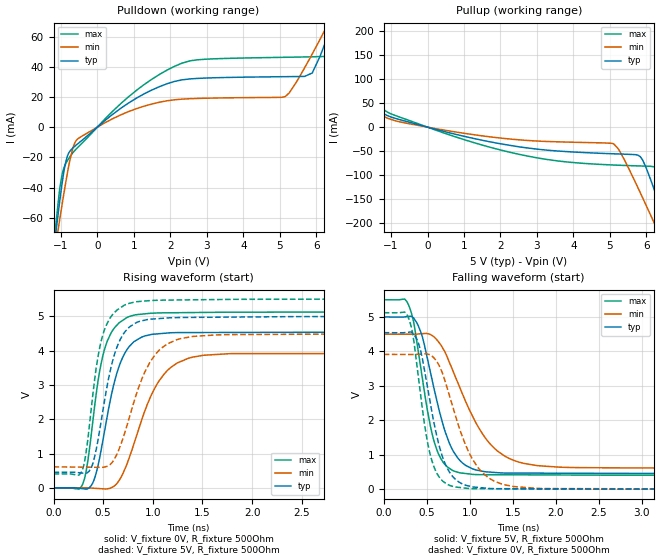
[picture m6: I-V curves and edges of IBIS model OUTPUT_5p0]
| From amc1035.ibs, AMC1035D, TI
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|   OUTPUT_5p0 Model
[Model]   OUTPUT_5p0
Model_type   Output
Polarity   Non-Inverting
Vmeas = 2.5
Vref = 0
Cref = 2pF
Rref = 100000
|   typ   min   max
C_comp   1.411E-12   1.379E-12   1.431E-12
|  Where Nom  PVT is Nominal Process,  5.0V,   27C
|   Fast PVT is Strong Process,   5.5V,   -40C
|   Slow PVT is Weak Process,   4.5V,   131C
[Voltage Range]   5   4.5   5.5
|Junction Temperature
[Temperature Range]   27   131   -40
[Pullup Reference]   5   4.5   5.5
[Pulldown Reference]   0   0   0
[Power Clamp Reference]   5   4.5   5.5
[GND Clamp Reference]   0   0   0
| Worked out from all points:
|   slope of the pulldown table from 0 to 0.75 V, typ, clamps not added: 52.7 ohm
|   slope of the pullup table from 0 to 0.75 V, typ, clamps not added: 51.4 ohm
|   falling waveform, V_fixture 5V, R_fixture 500Ohm: 20-80 % time 278ps typ, 454ps min, 209ps max; typ from 5 V to 0.453 V
|   rising waveform, V_fixture 0V, R_fixture 500Ohm: 20-80 % time 206ps typ, 316ps min, 164ps max; typ from 0 V to 4.54 V
|   rising waveform, V_fixture 5V, R_fixture 500Ohm: 20-80 % time 192ps typ, 292ps min, 153ps max; typ from 0.453 V to 5 V
|   falling waveform, V_fixture 0V, R_fixture 500Ohm: 20-80 % time 227ps typ, 341ps min, 178ps max; typ from 4.54 V to 0 V
[Pulldown]
|   Voltage   I(typ)   I(min)   I(max)
-5V       -944.3mA   -729.6mA   -1.186A
-1.25V    -93.96mA   -95.93mA   -94.24mA
-1.13V    -68.8mA    -76.76mA   -62.97mA
-920mV    -30.02mA   -44.54mA   -27.17mA
-545mV    -11.2mA    -7.985mA   -13.68mA
1.06V     19.03mA    12.14mA    24.13mA
2.32V     31.32mA    18.55mA    42.39mA
5.155V    33.43mA    20.36mA    46.27mA
5.89V     35.87mA    48.48mA    46.6mA
6.295V    59.03mA    67.14mA    46.92mA
6.925V    102.1mA    97.6mA     86.9mA
10V       331.2mA    257.4mA    402.2mA
[Pullup]
|   Voltage   I(typ)   I(min)   I(max)
-5V       273.2mA    192.3mA    382.4mA
-2.975V   137.3mA    98.99mA    189.2mA
-1.64V    50.03mA    39.3mA     65.18mA
-965mV    20.22mA    15.22mA    26.68mA
2.32V     -38.9mA    -25.27mA   -53.6mA
5.095V    -55.72mA   -34.94mA   -79.16mA
5.83V     -61.57mA   -136.9mA   -81.16mA
6.28V     -144.8mA   -211.6mA   -83.82mA
6.595V    -214.3mA   -264.6mA   -112.8mA
6.79V     -258mA     -297.6mA   -163.5mA
7.135V    -336mA     -356.1mA   -260.8mA
10V       -992.4mA   -846.3mA   -1.1A
[Ramp]
R_load = 500
|   typ   min   max
dV/dt_r   2.7263/2.05638e-10   2.34756/3.15181e-10   3.07412/1.63427e-10
dV/dt_f   2.72828/2.77617e-10   2.33315/4.53837e-10   3.05654/2.08549e-10
[Falling Waveform]
V_fixture = 5V
V_fixture_min = 4.5V
V_fixture_max = 5.5V
R_fixture = 500Ohm
C_fixture = 0F
|   Time   V(typ)   V(min)   V(max)
0s        5V         4.5V       5.5V
269.6ps   5.009V     4.498V     5.445V
380.5ps   4.85V      4.502V     4.352V
542ps     3.406V     4.491V     1.839V
638.3ps   2.354V     4.273V     1.014V
810.9ps   1.092V     3.396V     533.3mV
1.041ns   582.8mV    2.076V     427.6mV
1.456ns   466.9mV    895.1mV    417.8mV
2.229ns   462.2mV    626.8mV    410.2mV
45.47ns   452.9mV    611.4mV    405.8mV
[Rising Waveform]
V_fixture = 0V
V_fixture_min = 0V
V_fixture_max = 0V
R_fixture = 500Ohm
C_fixture = 0F
|   Time   V(typ)   V(min)   V(max)
0s        -77.83nV   -60.52nV   -192.2nV
277.8ps   -19.92mV   753.4uV    20.62mV
380.5ps   68.91mV    -6.155mV   1.566V
477.3ps   1.072V     -25.23mV   3.595V
577.2ps   2.631V     -1.867mV   4.5V
740.1ps   4.03V      700.6mV    4.964V
980.3ps   4.466V     2.674V     5.087V
1.245ns   4.523V     3.637V     5.103V
1.789ns   4.527V     3.912V     5.117V
45.47ns   4.544V     3.913V     5.124V
[Rising Waveform]
V_fixture = 5V
V_fixture_min = 4.5V
V_fixture_max = 5.5V
R_fixture = 500Ohm
C_fixture = 0F
|   Time   V(typ)   V(min)   V(max)
0s        452.8mV    611.4mV    405.7mV
294.3ps   429mV      603mV      555mV
380.5ps   587.9mV    600.6mV    2.32V
463ps     1.646V     598.3mV    4.06V
587.7ps   3.613V     729.4mV    5.021V
717.2ps   4.54V      1.603V     5.328V
980.3ps   4.915V     3.702V     5.458V
1.245ns   4.96V      4.319V     5.473V
1.789ns   4.974V     4.465V     5.491V
45.47ns   5V         4.5V       5.5V
[Falling Waveform]
|Gnd
V_fixture = 0V
V_fixture_min = 0V
V_fixture_max = 0V
R_fixture = 500Ohm
C_fixture = 0F
|   Time   V(typ)   V(min)   V(max)
0s        4.544V     3.913V     5.124V
303.5ps   4.561V     3.911V     4.858V
421.6ps   4.094V     3.921V     2.886V
509.4ps   2.956V     3.922V     1.362V
587.7ps   1.883V     3.802V     627.7mV
740.1ps   600mV      2.917V     138.7mV
980.3ps   96.77mV    1.123V     20.93mV
1.281ns   15.55mV    239.2mV    12.52mV
1.873ns   10.87mV    16.96mV    7.241mV
45.47ns   22.63uV    27.06uV    15.44uV
